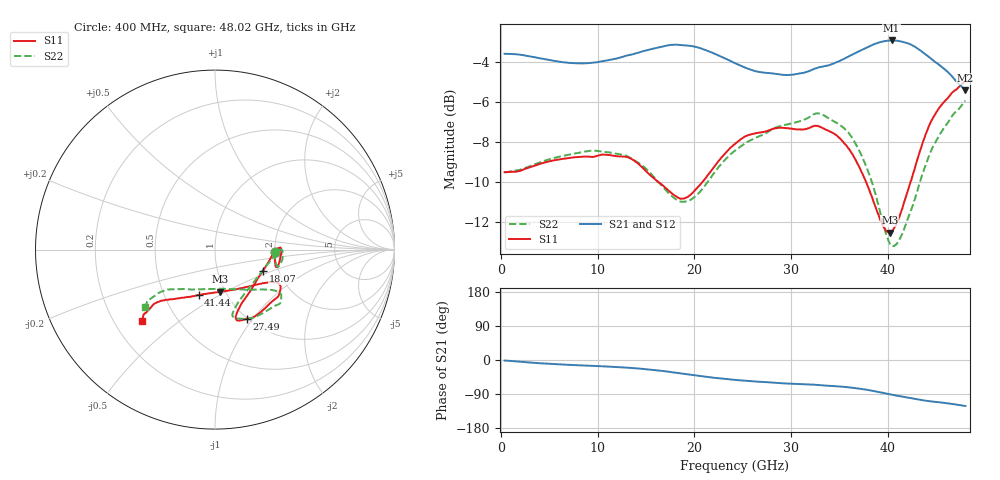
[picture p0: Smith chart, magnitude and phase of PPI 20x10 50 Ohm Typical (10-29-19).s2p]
!Keysight Technologies,N5227A,US56070614,A.10.47.06
!Date:	11/6/2019
!Correction
!S11(Full 2 Port(1,2))
!S21(Full 2 Port(1,2))
!S12(Full 2 Port(1,2))
!S22(Full 2 Port(1,2))
!S2P File: Measurements: S11, S21, S12, S22
# GHz S  dB  R 50
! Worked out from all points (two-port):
!   769 points, 400 MHz to 48.02 GHz, reference 50 ohm
!   highest |S21| = -2.90 dB at 40.39 GHz (marker M1); lowest = -5.4 dB at 48.02 GHz (marker M2)
!   |S21| within 3 dB of the highest: start of sweep to end of sweep
!   lowest |S11| = -12.5 dB at 40.2 GHz (marker M3), VSWR 1.62, Z = 47.2 - j23.5 ohm
!   |S11| at or under -10 dB: 16.31 GHz to 20.82 GHz (4.513 GHz wide, 24.3 % of centre); 37.77 GHz to 42.34 GHz (4.575 GHz wide, 11.4 % of centre)
!   |S22| runs from -13.2 to -5.9 dB; largest |S21 - S12| = 0.00071
!   S11 on the Smith chart (normalised r, x): 400 MHz: 2.01, -0.06; 18.07 GHz: 1.66, -0.43; 27.49 GHz: 0.99, -0.93; 41.44 GHz: 0.74, -0.40; 48.02 GHz: 0.32, -0.37
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0.4  -9.50 -2.3  -3.56 -1.4  -3.56 -1.4  -9.51 -2.5
4.43  -9.03 -15.9  -3.82 -9.2  -3.83 -9.2  -8.94 -15.0
8.34  -8.73 -8.8  -4.05 -14.3  -4.05 -14.2  -8.50 -10.5
12.61  -8.71 1.5  -3.71 -19.3  -3.72 -19.3  -8.63 0.3
14.54  -9.22 0.6  -3.46 -23.1  -3.46 -23.1  -9.14 -1.6
16.33  -10.01 -7.6  -3.25 -27.8  -3.25 -27.8  -10.02 -11.2
18.07  -10.69 -24.1  -3.11 -33.5  -3.11 -33.5  -10.85 -27.3
19.56  -10.65 -42.6  -3.17 -38.7  -3.17 -38.7  -10.90 -46.7
21.54  -9.56 -63.1  -3.44 -45.4  -3.45 -45.4  -9.88 -66.1
24.21  -8.08 -73.0  -4.03 -52.5  -4.04 -52.5  -8.42 -75.2
27.49  -7.44 -65.6  -4.52 -58.5  -4.52 -58.5  -7.52 -65.7
29.11  -7.27 -58.0  -4.62 -61.5  -4.62 -61.5  -7.16 -57.9
32.21  -7.21 -38.3  -4.36 -64.8  -4.36 -64.8  -6.63 -41.1
34.38  -7.55 -29.4  -4.06 -68.7  -4.06 -68.6  -6.94 -34.9
36.3  -8.56 -29.0  -3.61 -73.1  -3.62 -73.1  -7.77 -34.1
38.16  -10.50 -41.0  -3.17 -79.9  -3.18 -79.9  -9.71 -42.9
40.14  -12.51 -81.6  -2.90 -90.2  -2.91 -90.2  -12.99 -77.6
40.2  -12.53 -83.3  -2.90 -90.5  -2.91 -90.5  -13.08 -79.2
40.39  -12.45 -88.1  -2.90 -91.5  -2.90 -91.5  -13.17 -84.3
41.44  -11.40 -109.8  -2.96 -96.4  -2.96 -96.4  -12.65 -108.9
44.42  -7.01 -138.0  -3.79 -109.2  -3.80 -109.2  -8.48 -141.8
48.02  -4.92 -135.9  -5.40 -121.4  -5.41 -121.4  -5.92 -140.7
